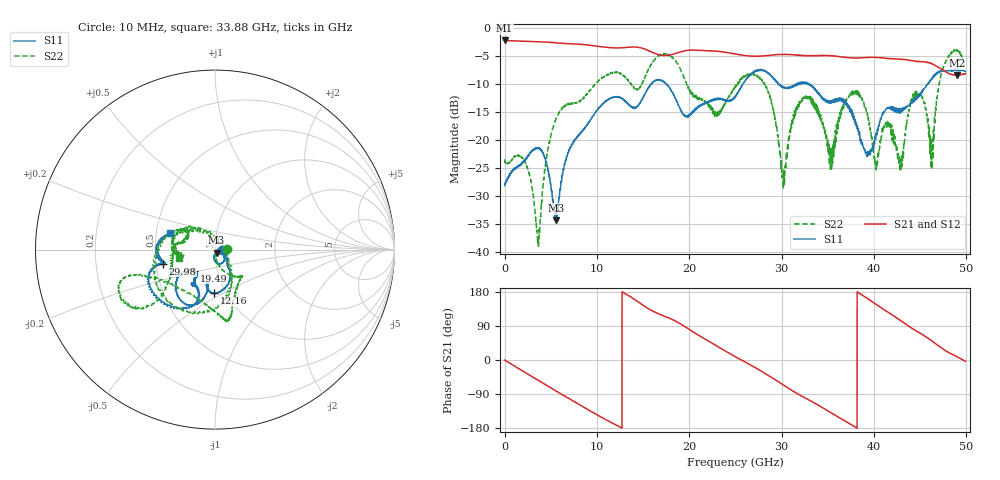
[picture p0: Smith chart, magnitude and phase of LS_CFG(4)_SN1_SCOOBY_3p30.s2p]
!Keysight Technologies,N5245B,MY58422026,A.13.80.08
!Date: Thursday, March 19, 2020 23:27:52
!Correction: S11(Full 2 Port(1,2))
!S21(Full 2 Port(1,2))
!S12(Full 2 Port(1,2))
!S22(Full 2 Port(1,2))
!S2P File: Measurements: S11, S21, S12, S22:
# Hz S DB R 50.0
!freq dBS11 angS11 dBS21 angS21 dBS12 angS12 dBS22 angS22
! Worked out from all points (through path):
!   4991 points, 10 MHz to 49.91 GHz, reference 50 ohm
!   highest |S21| = -2.22 dB at 10 MHz (marker M1); lowest = -8.4 dB at 49.01 GHz (marker M2)
!   group delay of S21, straight-line fit = 39.9 ps
!   lowest |S11| = -34.3 dB at 5.55 GHz (marker M3), VSWR 1.04, Z = 50.8 - j1.77 ohm
!   |S11| at or under -10 dB: start of sweep to 15.84 GHz; 17.55 GHz to 25.81 GHz (8.261 GHz wide, 38.1 % of centre); 33.06 GHz to 45.8 GHz (12.73 GHz wide, 32.3 % of centre)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
!   |S22| runs from -38.9 to -3.8 dB; largest |S21 - S12| = 0.0071
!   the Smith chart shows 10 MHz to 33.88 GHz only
!   S11 on the Smith chart (normalised r, x): 10 MHz: 1.08, -0.01; 12.16 GHz: 0.88, -0.45; 19.49 GHz: 0.77, -0.18; 29.98 GHz: 0.55, -0.09; 33.88 GHz: 0.59, +0.12
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1e7  -28.09 -4.9  -2.22 -0.3  -2.21 -0.3  -23.40 1.7
2.25e9  -23.39 -39.5  -2.37 -33.2  -2.36 -33.2  -23.87 0.5
3.63e9  -21.44 -65.7  -2.45 -53.2  -2.44 -53.2  -37.46 -26.3
5.55e9  -34.27 -63.9  -2.63 -81.4  -2.63 -81.4  -16.28 -62.6
8.33e9  -18.64 -52.0  -2.92 -120.9  -2.92 -120.9  -12.80 -54.7
1.216e10  -12.31 -91.5  -3.55 -172.6  -3.54 -172.6  -7.90 -81.2
1.665e10  -9.26 -119.0  -4.73 122.1  -4.73 122.2  -5.03 -160.5
1.949e10  -15.64 -135.1  -4.08 88.9  -4.07 88.9  -9.07 -141.2
2.496e10  -12.36 -113.3  -4.60 9.3  -4.59 9.4  -10.66 172.5
2.817e10  -7.69 -153.1  -4.96 -34.6  -4.96 -34.6  -10.03 -86.5
2.998e10  -10.50 -164.9  -4.72 -62.5  -4.72 -62.4  -23.59 -8.3
3.328e10  -10.27 167.8  -4.94 -110.0  -4.94 -109.7  -12.80 -176.8
3.388e10  -11.38 159.2  -4.95 -118.2  -4.95 -117.8  -14.07 -165.9
3.541e10  -13.27 137.0  -4.93 -139.9  -4.89 -139.6  -25.23 164.5
3.929e10  -22.40 98.0  -5.26 162.5  -5.24 162.3  -15.14 -132.1
4.023e10  -18.99 67.7  -5.24 146.9  -5.22 146.5  -25.26 -37.4
4.16e10  -14.11 44.3  -5.45 125.1  -5.47 124.9  -17.15 72.1
4.295e10  -14.95 33.4  -5.58 103.3  -5.61 103.2  -25.15 27.2
4.492e10  -11.76 -9.0  -5.96 72.2  -5.98 72.1  -11.81 17.8
4.627e10  -8.91 -15.4  -6.34 50.5  -6.36 50.4  -24.87 -33.1
4.901e10  -7.30 -47.0  -8.41 8.4  -8.42 8.3  -3.84 -46.1
4.991e10  -7.75 -43.7  -8.14 -3.4  -8.17 -3.5  -6.64 -27.4
